PROGRAM EL6001_MASTER
VAR
   Timer: TON; // Timer for periodical requests by the master
   Send: SendData; // Functionblock of TC2_SerialCom
   SendBusy: BOOL; // Flag copy of SendData.Busy
   SendErrorID: ComError_t; // Flag-Copy of Error-ID
   aDataTX:tDataFrame; // Data frame being send
   Receive: ReceiveData; // Functionblock of TC2_SerialCom
   LastReceivedDataBytes: tDataFrame; // Copy (Latch) of received data
   DataReceived: BOOL; // Flag copy of receive confirmation
   ReceiveBusy: BOOL; // Flag copy of reception not ready
   ReceiveError: BOOL; // Flag copy of receive error
   ReceiveErrorID: ComError_t;// Error-ID copy
   ReceiveTimeout: BOOL; // Flag copy of receive-timeout
   ReceiveCounter: UDINT := 0; // Number of received frames
   aDataRX:tDataFrame; // Receiving data frame buffer
   nDataLen:BYTE := 4; // Fixed data length
   nState:BYTE := 0; // Initial state (start)
   bNodeId_SL1: BYTE := 16#07; // ID of slave node
   bReqLen_SL1: BYTE := 0; // Optional entry for 4 Data bytes Value 2
   nRxChecksum: BYTE; // Storage of received checksum
   nCalcChecksum:BYTE; // Storage of calculated checksum
   T_ReceiveDelay:TIME; // Storage of calculated delay time
END_VAR

(*==================================================================
Receive data
*)
CASE nState OF
0:
   Timer(IN:=TRUE, PT:=T#0.5S); // Call timer for periodical master requests
   IF Timer.Q THEN
      // Put ID into Tranceive data:
      aDataTX[0] := F_ADD_LIN_NODE_PARITY(bNodeId_SL1, bReqLen_SL1);
      LastReceivedDataBytes[0] := aDataTX[0];
      // Send request to Slave 1 (get Data)
      Send(pSendData:= ADR(aDataTX), Length:= 1,
      TXbuffer:= TxBuffer_MASTER,
      Busy => SendBusy, Error => SendErrorID);
      Timer(IN:=FALSE); (* reset timer *)
      IF NOT SendBusy THEN // Wait until sending ends
      nState := nState + 1;
      END_IF
   END_IF
1:
   // Delaytime by 1/Tbaud * Number of Bytes * (8 Databits + 2 Bit:start-Stop) * 1000ms
   T_ReceiveDelay := REAL_TO_TIME((1/DINT_TO_REAL(nSetBaudrate)) * 33 * 1000); // .. for 1 Byte
   Timer(IN:=TRUE, PT:=T_ReceiveDelay);
   IF Timer.Q THEN
      // Wait until ID is send
      nState := nState + 1;
      Timer(IN:=FALSE); (* reset timer *)
   END_IF
2:
   Receive(
   pReceiveData:= ADR(aDataRX),
   SizeReceiveData:= (nDataLen + 1),
   RXbuffer:= RxBuffer_MASTER,
   Timeout:= T#1S,
   DataReceived=> DataReceived,
   busy=> ReceiveBusy,
   Error=> ReceiveErrorID,
   RxTimeout=> ReceiveTimeout );
   IF DataReceived THEN
      // DataReceived := FALSE;
      ReceiveCounter := ReceiveCounter + 1;
      IF NOT ReceiveBusy THEN
         // Compare checksum
         nRxChecksum := aDataRX[nDataLen];
         nCalcChecksum := F_CALC_LIN_CHKSUM(pData := ADR(aDataRX), nLen := nDataLen);
         IF(nRxChecksum = nCalcChecksum) THEN
            // Response received - clear databuffer:
            memset(ADR(LastReceivedDataBytes[1]), 0, (SIZEOF(aDataRX)-1));
            // Take-over data when checksum OK:
            memcpy(ADR(LastReceivedDataBytes[1]), ADR(aDataRX), (nDataLen +1));
         END_IF
      nState := 0;
      END_IF
   ELSE
      Timer(IN:=TRUE, PT:=T#0.1S); // Receive-Timeout 100 ms: no data
      IF Timer.Q THEN
         nState := 0;
      END_IF
   END_IF
END_CASE
(*==================================================================
*)

END_PROGRAM
